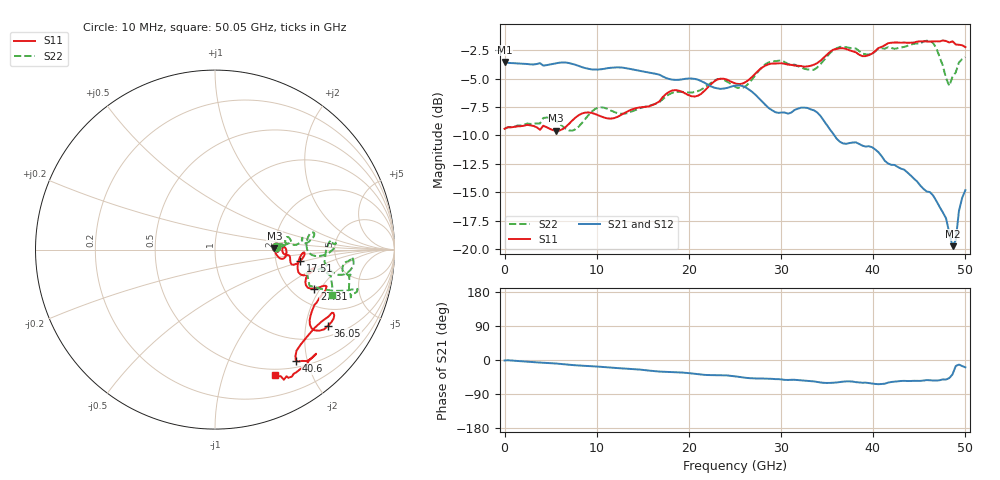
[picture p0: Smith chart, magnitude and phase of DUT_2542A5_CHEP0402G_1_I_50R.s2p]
! 11/3/2025 4:08:25 PM
! C:\MESURES\046-TRL-DUT-CHEP\0402\DUT-2542A5-CHEP0402G-1-I.S2P
! CHANNEL.1 Sparams
! TR.MEASUREMENT
! CORRECTED.DATA
! RF.CORRECTION: CAL.A: FULL.TWO.PORT.CALCAL.A: Port 1,4
! AVERAGING.OFF
! IF.BANDWIDTH: 500HZ
! SWEEPTYPE:  FREQ.SWEEP(Linear)
! Reference Plane Port Info
! PORT:  PORT1  PORT4
! DISTANCE:  0  m  0  m
! TIME:  0  s  0  s
! PHASE.OFFSET:  0  deg.  0  deg.
! LOSS:  0  dB  0  dB
! REF.LOSS:  0  dB  0  dB
! REF.FREQ:  0  Hz  0  Hz
! Power Info
! POWER:  -10  dBm  -10  dBm
! EFF.POWER:  -10  dBm  -10  dBm
! SOURCE.ATTEN:  0  dB  0  dB
! TEST.ATTEN:  0  dB  0  dB
! PORTZ: Port1:50 Port4:50
# GHZ S RI R 50
! FREQ.GHZ  S11RE  S11IM  S41RE  S41IM  S14RE  S14IM  S44RE  S44IM
!; PortSelection: Port_14 (1-->1,4-->4)
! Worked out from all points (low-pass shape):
!   144 points, 10 MHz to 50.05 GHz, reference 50 ohm
!   highest |S21| = -3.55 dB at 10 MHz (marker M1); lowest = -19.8 dB at 48.65 GHz (marker M2)
!   |S21| within 3 dB of the highest: start of sweep to 27.41 GHz
!   lowest |S11| = -9.6 dB at 5.609 GHz (marker M3), VSWR 1.99, Z = 99.5 + j2.07 ohm
!   |S11| at or under -10 dB: nowhere
!   |S22| runs from -9.6 to -1.7 dB; largest |S21 - S12| = 0.0028
!   S11 on the Smith chart (normalised r, x): 10 MHz: 2.02, +0.07; 17.51 GHz: 2.76, -0.46; 27.31 GHz: 2.63, -1.76; 36.05 GHz: 1.34, -2.68; 40.6 GHz: 0.60, -1.81; 50.05 GHz: 0.43, -1.50
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0.01  0.3376 0.0155  0.6643 -0.0142  0.6643 -0.015  0.3377 0.0155
5.6092  0.331 0.00925  0.648 -0.106  0.6469 -0.1047  0.3642 0.0309
8.4088  0.3927 -0.0402  0.6095 -0.1638  0.6088 -0.1618  0.3581 0.00976
10.5085  0.3824 0.0153  0.5877 -0.1909  0.5871 -0.189  0.4183 0.039
16.8076  0.4375 -0.0847  0.5038 -0.2973  0.5043 -0.2946  0.4412 0.0255
17.5075  0.4753 -0.0643  0.4841 -0.2938  0.4847 -0.2925  0.4666 0.0341
19.25725  0.4918 -0.0166  0.4672 -0.3039  0.4683 -0.3019  0.4869 0.0661
21.7069  0.4764 -0.139  0.418 -0.3409  0.4193 -0.3397  0.5117 0.0374
25.2064  0.5144 -0.1404  0.3793 -0.362  0.3802 -0.3613  0.5109 0.0476
27.3061  0.5541 -0.2168  0.3135 -0.3565  0.315 -0.3552  0.5853 -0.0353
29.05585  0.6217 -0.2055  0.2635 -0.3113  0.2651 -0.3104  0.6692 0.0194
31.5055  0.5829 -0.2678  0.2505 -0.3234  0.2517 -0.3227  0.6458 0.0506
33.6052  0.5323 -0.3677  0.2249 -0.3397  0.2262 -0.3399  0.6103 -0.0687
36.05485  0.6304 -0.4231  0.1562 -0.2634  0.1558 -0.2632  0.755 -0.1134
37.8046  0.6522 -0.3517  0.1604 -0.2464  0.1605 -0.2456  0.7635 -0.0415
40.6042  0.4503 -0.6195  0.1176 -0.2394  0.1174 -0.239  0.7482 -0.1477
42.004  0.5274 -0.6125  0.1242 -0.199  0.1247 -0.1975  0.7533 -0.1422
44.8036  0.5126 -0.6363  0.1137 -0.1623  0.1139 -0.1612  0.7566 -0.2662
46.2034  0.4758 -0.6654  0.1057 -0.1432  0.106 -0.1414  0.795 -0.2191
47.95315  0.4082 -0.7143  0.0848 -0.1067  0.0855 -0.1051  0.5268 -0.2013
48.65305  0.3835 -0.725  0.0809 -0.0635  0.0808 -0.063  0.5594 -0.1186
50.05285  0.3322 -0.6981  0.1712 -0.0601  0.1719 -0.0588  0.6505 -0.2549
